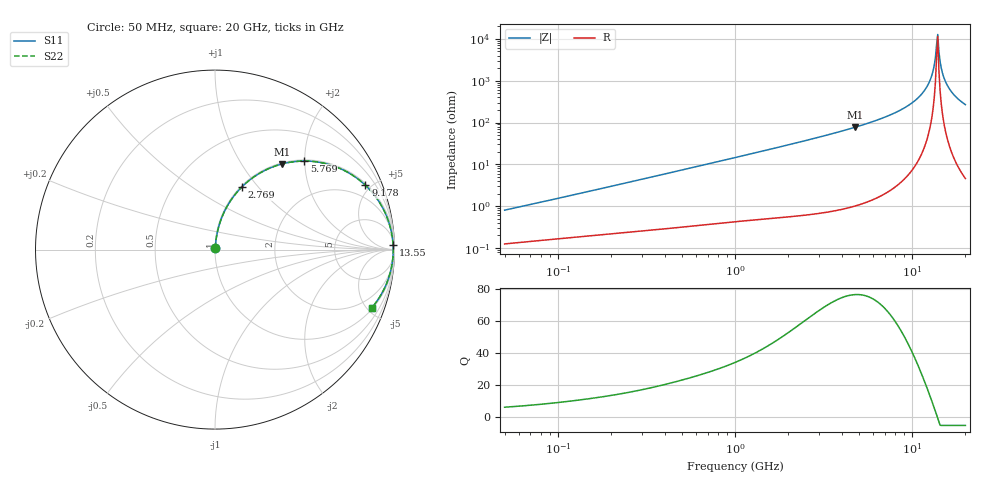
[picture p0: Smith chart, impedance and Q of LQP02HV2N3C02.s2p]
!Murata Part Number: LQP02HV2N3C02
!These Parameters are Measured in Series Mode Connection
!  o--[Z]--o
!Port1  Port2
!  o-------o
!Freq. Start=50[MHz] Stop=20[GHz], 401[Steps]
# Hz S RI R 50
!Freq.(Hz) S11(Real) S11(Imag) S21(Real) S21(Imag) S12(Real) S12(Imag) S22(Real) S22(Imag)
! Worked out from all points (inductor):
!   401 points, 50 MHz to 20 GHz, reference 50 ohm
!   read as one part in series: L = 2.49 nH near 51.52 MHz
!   highest Q = 76.4 at 4.748 GHz (marker M1), where L = 2.57 nH
!   self-resonance near 13.75 GHz
!   S11 on the Smith chart (normalised r, x): 50 MHz: 1.00, +0.02; 2.769 GHz: 1.01, +0.82; 5.769 GHz: 1.03, +1.99; 9.178 GHz: 1.09, +4.64; 13.55 GHz: 20, +70; 20 GHz: 1.09, -5.35
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5e7  0.00131 0.00792  0.9987 -0.00792  0.9987 -0.00792  0.00131 0.00792
1.364002e8  0.00229 0.0205  0.9977 -0.0205  0.9977 -0.0205  0.00229 0.0205
3.721004e8  0.00573 0.0542  0.9943 -0.0542  0.9943 -0.0542  0.00573 0.0542
1e9  0.0246 0.1409  0.9754 -0.1409  0.9754 -0.1409  0.0246 0.1409
2.728004e9  0.1453 0.3446  0.8547 -0.3446  0.8547 -0.3446  0.1453 0.3446
2.769174e9  0.1493 0.3486  0.8507 -0.3486  0.8507 -0.3486  0.1493 0.3486
4.748272e9  0.3724 0.4769  0.6276 -0.4769  0.6276 -0.4769  0.3724 0.4769
5.769027e9  0.4975 0.4933  0.5025 -0.4933  0.5025 -0.4933  0.4975 0.4933
7.442007e9  0.6863 0.4563  0.3137 -0.4563  0.3137 -0.4563  0.6863 0.4563
9.178299e9  0.8382 0.3582  0.1618 -0.3582  0.1618 -0.3582  0.8382 0.3582
1.082228e10  0.9321 0.2364  0.0679 -0.2364  0.0679 -0.2364  0.9321 0.2364
1.201863e10  0.9716 0.1427  0.0284 -0.1427  0.0284 -0.1427  0.9716 0.1427
1.295331e10  0.9877 0.0707  0.0123 -0.0707  0.0123 -0.0707  0.9877 0.0707
1.314879e10  0.9896 0.056  0.0104 -0.056  0.0104 -0.056  0.9896 0.056
1.354865e10  0.9922 0.0264  0.00781 -0.0264  0.00781 -0.0264  0.9922 0.0264
1.375312e10  0.9928 0.0115  0.0072 -0.0115  0.0072 -0.0115  0.9928 0.0115
1.417136e10  0.9927 -0.0182  0.00732 0.0182  0.00732 0.0182  0.9927 -0.0182
1.460232e10  0.9908 -0.0479  0.00923 0.0479  0.00923 0.0479  0.9908 -0.0479
1.504638e10  0.9871 -0.0774  0.0129 0.0774  0.0129 0.0774  0.9871 -0.0774
1.621653e10  0.9704 -0.1492  0.0296 0.1492  0.0296 0.1492  0.9704 -0.1492
1.774144e10  0.937 -0.2301  0.063 0.2301  0.063 0.2301  0.937 -0.2301
2e10  0.8734 -0.3241  0.1266 0.3241  0.1266 0.3241  0.8734 -0.3241
